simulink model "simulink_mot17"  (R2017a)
settings: Solver=VariableStepAuto  StartTime=0.0  StopTime=1  MaxStep=0.0001  RelTol=1e-5
undefined symbols (not defined in the file or in its folder): j

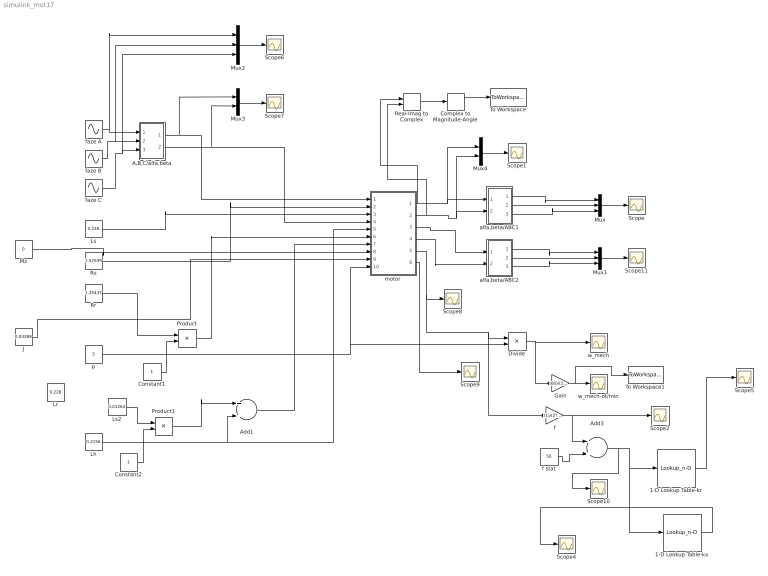
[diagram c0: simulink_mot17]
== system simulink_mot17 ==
  1-D Lookup Table-kr : Lookup_n-D  NumberOfTableDimensions=1  BreakpointsForDimension1="[0\t1.02040816326531\t2.04081632653061\t3.06122448979592\t4.08163265306123\t5.10204081632653\t6.12244897959184\t7.14285714285714\t8.16326530612245\t9.18367346938776\t10.2040816326531\t11.2244897959184\t12.2448979591837\t13.2653061224490\t14.2857142857143\t15.3061224489796\t16.3265306122449\t17.3469387755102\t18.3673469387755\t19.3877551020408\t20.4081632653061\t21.4285714285714\t22.4489795918367\t23.4693877551020\t24.489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"  Table="[1.00000000000000\t1.00003541196316\t1.00014163999465\t1.00031866052521\t1.00056643428835\t1.00088490634371\t1.00127400610982\t1.00173364740605\t1.00226372850387\t1.00286413218725\t1.00353472582216\t1.00427536143518\t1.00508587580093\t1.00596609053850\t1.00691581221651\t1.00793483246685\t1.00902292810692\t1.01017986127023\t1.01140537954524\t1.01269921612228\t1.01406108994838\t1.01549070588984\t1.01698775490243\t1.018551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"  InternalRulePriority=Speed  RndMeth=Simplest
  1-D Lookup Table-kx : Lookup_n-D  NumberOfTableDimensions=1  BreakpointsForDimension1="[0\t1.02040816326531\t2.04081632653061\t3.06122448979592\t4.08163265306123\t5.10204081632653\t6.12244897959184\t7.14285714285714\t8.16326530612245\t9.18367346938776\t10.2040816326531\t11.2244897959184\t12.2448979591837\t13.2653061224490\t14.2857142857143\t15.3061224489796\t16.3265306122449\t17.3469387755102\t18.3673469387755\t19.3877551020408\t20.4081632653061\t21.4285714285714\t22.4489795918367\t23.4693877551020\t24.489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"  Table="[1.00000000000000\t0.999988691005197\t0.999954766683005\t0.999898235018478\t0.999819109314739\t0.999717408185028\t0.999593155541589\t0.999446380581399\t0.999277117768758\t0.999085406814764\t0.998871292653684\t0.998634825416263\t0.998376060399988\t0.998095058036341\t0.997791883855089\t0.997466608445635\t0.997119307415473\t0.996750061345821\t0.996358955744429\t0.995946080995662\t0.995511532307881\t0.995055409658204\t0.99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"  InternalRulePriority=Speed  RndMeth=Simplest
  A,B,C/alfa,beta : Subsystem
  Add1 : Sum
  Add3 : Sum  Inputs=-+
  Complex to Magnitude-Angle : ComplexToMagnitudeAngle
  Constant1 : Constant
  Constant2 : Constant
  Divide : Product  Inputs=*/
  Gain : Gain  Gain=(60)/(2*pi)
  J : Constant  Value=0.03389
  Lh : Constant  Value=0.2156
  Lr : Constant  Value=0.228
  Ls : Constant  Value=0.226
  Ls2 : Constant  Value=0.01264
  Mux : Mux  Inputs=3
  Mux1 : Mux  Inputs=3
  Mux2 : Mux  Inputs=3
  Mux3 : Mux  Inputs=2
  Mux4 : Mux  Inputs=2
  Mz : Constant  Value=0
  Product : Product
  Product1 : Product
  Real-Imag to Complex : RealImagToComplex
  Rr : Constant  Value=1.35437
  Rs : Constant  Value=1.52939
  Scope{,1..2,4..11} (11 alike) : Scope
  To Workspace : ToWorkspace  VariableName=Istat  SampleTime=-1
  To Workspace1 : ToWorkspace  VariableName=ot  SampleTime=-1
  alfa,beta/ABC1 : Subsystem
  alfa,beta/ABC2 : Subsystem
  f : Gain  Gain=(1)/(2*pi)
  f stat : Constant  Value=50
  faze A : Sin  Amplitude=230*1.41421356237309  Frequency=314.159265  SampleTime=0
  faze B : Sin  Amplitude=230*1.41421356237309  Frequency=314.159265  Phase=-(2*pi/3)  SampleTime=0
  faze C : Sin  Amplitude=230*1.41421356237309  Frequency=314.159265  Phase=(2*pi/3)  SampleTime=0
  motor : Subsystem
  p : Constant  Value=3
  w_mech : Scope
  w_mech-ot/min : Scope
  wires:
  faze A/1 -> Mux2/1, A,B,C/alfa,beta/1(In1)
  faze B/1 -> Mux2/2, A,B,C/alfa,beta/2(In2)
  faze C/1 -> Mux2/3, A,B,C/alfa,beta/3(In3)
  A,B,C/alfa,beta/1(Out1) -> Mux3/1, motor/1(Us_alfa)
  Rs/1 -> motor/2(Rs)
  Ls/1 -> motor/3(Ls)
  Lh/1 -> Add1/2, motor/5(Lh)
  motor/3(Ir_alfa1) -> alfa,beta/ABC2/1(Ir_alfa)
  motor/4(Ir_beta) -> alfa,beta/ABC2/2(Ir_beta)
  motor/1(Is_alfa) -> Real-Imag to Complex/1, Mux4/1, alfa,beta/ABC1/1(Is_alfa)
  motor/2(Is_beta) -> Real-Imag to Complex/2, Mux4/2, alfa,beta/ABC1/2(Is_beta)
  A,B,C/alfa,beta/2(Out2) -> Mux3/2, motor/4(Us beta)
  alfa,beta/ABC1/2(Out2) -> Mux/2
  alfa,beta/ABC1/3(Out3) -> Mux/3
  alfa,beta/ABC2/1(Out1) -> Mux1/1
  alfa,beta/ABC2/2(Out2) -> Mux1/2
  alfa,beta/ABC2/3(Out3) -> Mux1/3
  p/1 -> Divide/2, motor/10(p)
  Mz/1 -> motor/8(Mz)
  J/1 -> motor/9(J)
  motor/5(w_el) -> Scope8/1, f/1, Divide/1
  motor/6(M_elmag1) -> Scope9/1
  Divide/1 -> Gain/1, w_mech/1
  alfa,beta/ABC1/1(Out1) -> Mux/1
  Mux/1 -> Scope/1
  Mux1/1 -> Scope11/1
  Mux2/1 -> Scope6/1
  Mux3/1 -> Scope7/1
  Mux4/1 -> Scope1/1
  Gain/1 -> To Workspace1/1, w_mech-ot/min/1
  f stat/1 -> Add3/2
  f/1 -> Scope2/1, Add3/1
  Add3/1 -> Scope10/1, 1-D Lookup Table-kx/1, 1-D Lookup Table-kr/1
  1-D Lookup Table-kr/1 -> Scope5/1
  Rr/1 -> Product/1
  Product/1 -> motor/6(Rr)
  Real-Imag to Complex/1 -> Complex to Magnitude-Angle/1
  Complex to Magnitude-Angle/1 -> To Workspace/1
  Ls2/1 -> Product1/1
  Product1/1 -> Add1/1
  Add1/1 -> motor/7(Lr)
  1-D Lookup Table-kx/1 -> Scope4/1
  Constant2/1 -> Product1/2
  Constant1/1 -> Product/2

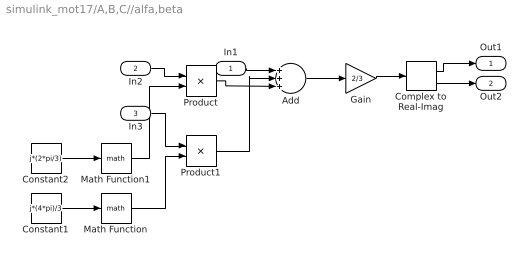
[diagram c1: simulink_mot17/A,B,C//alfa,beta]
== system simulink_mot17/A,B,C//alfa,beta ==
  In1 : Inport
  In2 : Inport  Port=2
  In3 : Inport  Port=3
  Add : Sum  Inputs=+++
  Complex to Real-Imag : ComplexToRealImag
  Constant1 : Constant  Value=j*(4*pi)/3
  Constant2 : Constant  Value=j*(2*pi/3)
  Gain : Gain  Gain=2/3
  Math Function : Math
  Math Function1 : Math
  Product : Product
  Product1 : Product
  Out1 : Outport
  Out2 : Outport  Port=2
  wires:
  Math Function/1 -> Product1/2
  Product1/1 -> Add/2
  Add/1 -> Gain/1
  Constant1/1 -> Math Function/1
  Product/1 -> Add/3
  Complex to Real-Imag/2 -> Out2/1
  Gain/1 -> Complex to Real-Imag/1
  Math Function1/1 -> Product/2
  In3/1 -> Product1/1
  Complex to Real-Imag/1 -> Out1/1
  Constant2/1 -> Math Function1/1
  In1/1 -> Add/1
  In2/1 -> Product/1

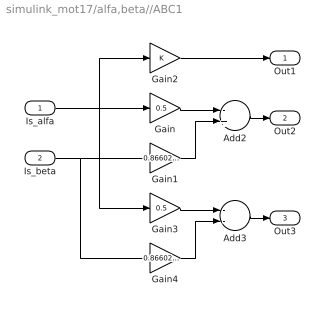
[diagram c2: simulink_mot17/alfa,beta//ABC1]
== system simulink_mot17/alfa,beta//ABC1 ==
  Is_alfa : Inport
  Is_beta : Inport  Port=2
  Add2 : Sum  Inputs=-+
  Add3 : Sum  Inputs=--
  Gain : Gain  Gain=0.5
  Gain1 : Gain  Gain=0.8660254037844
  Gain2 : Gain
  Gain3 : Gain  Gain=0.5
  Gain4 : Gain  Gain=0.8660254037844
  Out1 : Outport
  Out2 : Outport  Port=2
  Out3 : Outport  Port=3
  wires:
  Gain/1 -> Add2/1
  Is_alfa/1 -> Gain3/1, Gain2/1, Gain/1
  Gain4/1 -> Add3/2
  Gain1/1 -> Add2/2
  Is_beta/1 -> Gain4/1, Gain1/1
  Gain3/1 -> Add3/1
  Add2/1 -> Out2/1
  Add3/1 -> Out3/1
  Gain2/1 -> Out1/1

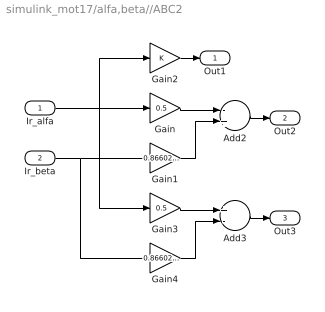
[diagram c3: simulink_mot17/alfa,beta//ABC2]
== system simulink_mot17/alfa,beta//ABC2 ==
  Ir_alfa : Inport
  Ir_beta : Inport  Port=2
  Add2 : Sum  Inputs=-+
  Add3 : Sum  Inputs=+-
  Gain : Gain  Gain=0.5
  Gain1 : Gain  Gain=0.8660254037844
  Gain2 : Gain
  Gain3 : Gain  Gain=0.5
  Gain4 : Gain  Gain=0.8660254037844
  Out1 : Outport
  Out2 : Outport  Port=2
  Out3 : Outport  Port=3
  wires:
  Gain/1 -> Add2/1
  Ir_alfa/1 -> Gain3/1, Gain2/1, Gain/1
  Gain4/1 -> Add3/2
  Gain1/1 -> Add2/2
  Ir_beta/1 -> Gain4/1, Gain1/1
  Gain3/1 -> Add3/1
  Add2/1 -> Out2/1
  Add3/1 -> Out3/1
  Gain2/1 -> Out1/1

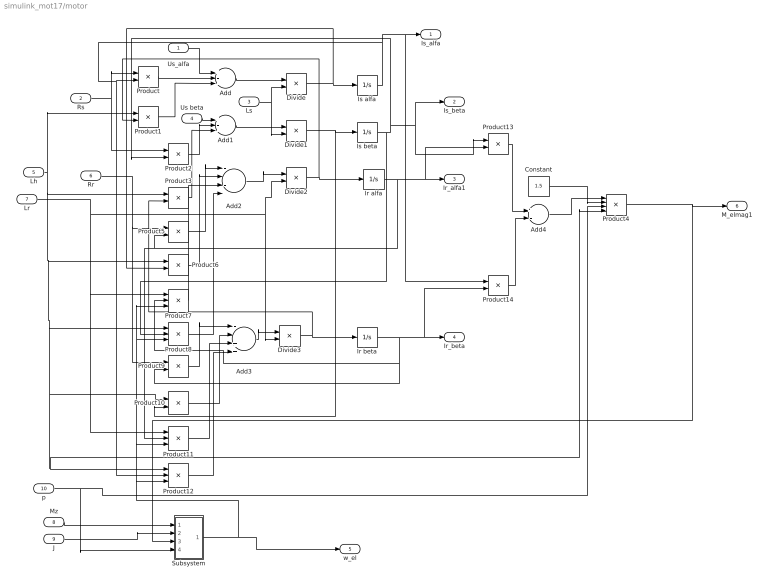
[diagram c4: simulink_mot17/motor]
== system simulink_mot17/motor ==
  Us_alfa : Inport
  Rs : Inport  Port=2
  Ls : Inport  Port=3
  Us beta : Inport  Port=4
  Lh : Inport  Port=5
  Rr : Inport  Port=6
  Lr : Inport  Port=7
  Mz : Inport  Port=8
  J : Inport  Port=9
  p : Inport  Port=10
  Add : Sum  Inputs=+--
  Add1 : Sum  Inputs=+--
  Add2 : Sum  Inputs=----
  Add3 : Sum  Inputs=--++
  Add4 : Sum  Inputs=+-
  Constant : Constant  Value=1.5
  Divide{,1..3} (4 alike) : Product  Inputs=*/
  Ir alfa : Integrator
  Ir beta : Integrator
  Is alfa : Integrator
  Is beta : Integrator
  Product{,1..3,5..6,9..10,13..14} (10 alike) : Product
  Product{7..8,11..12} (4 alike) : Product  Inputs=3
  Product4 : Product  Inputs=4
  Subsystem : Subsystem
  Is_alfa : Outport
  Is_beta : Outport  Port=2
  Ir_alfa1 : Outport  Port=3
  Ir_beta : Outport  Port=4
  w_el : Outport  Port=5
  M_elmag1 : Outport  Port=6
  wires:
  Lh/1 -> Product4/4, Product12/1, Product10/1, Product8/1, Product6/1, Product3/1, Product1/1
  Product6/1 -> Add2/2
  Product8/1 -> Add2/4
  Ir alfa/1 -> Product13/2, Ir_alfa1/1, Product11/2, Product5/2
  Product7/1 -> Add2/3
  Rs/1 -> Product2/1, Product/1
  Product1/1 -> Add/3
  Product/1 -> Add/2
  Is beta/1 -> Is_beta/1, Product13/1, Product2/2, Product8/2
  Ls/1 -> Divide1/2, Divide/2
  Add1/1 -> Divide1/1
  Divide2/1 -> Ir alfa/1, Product1/2
  Add/1 -> Divide/1
  Is alfa/1 -> Product14/1, Is_alfa/1, Product12/2, Product/2
  Product3/1 -> Add1/3
  Add2/1 -> Divide2/1
  Product5/1 -> Add2/1
  Rr/1 -> Product9/1, Product5/1
  Lr/1 -> Product11/1, Product7/1, Divide2/2, Divide3/2
  Product2/1 -> Add1/2
  Us beta/1 -> Add1/1
  Us_alfa/1 -> Add/1
  Product10/1 -> Add3/2
  Product11/1 -> Add3/3
  Divide3/1 -> Ir beta/1, Product3/2
  Product12/1 -> Add3/4
  Divide/1 -> Product6/2, Is alfa/1
  Divide1/1 -> Product10/2, Is beta/1
  Product9/1 -> Add3/1
  Add3/1 -> Divide3/1
  Mz/1 -> Subsystem/1(Mz)
  J/1 -> Subsystem/2(J)
  p/1 -> Subsystem/4(p), Product4/3
  Subsystem/1(Out1) -> Product12/3, Product11/3, Product8/3, Product7/3, w_el/1
  Ir beta/1 -> Product14/2, Ir_beta/1, Product9/2, Product7/2
  Product13/1 -> Add4/1
  Product14/1 -> Add4/2
  Add4/1 -> Product4/1
  Constant/1 -> Product4/2
  Product4/1 -> Subsystem/3(Melmag), M_elmag1/1

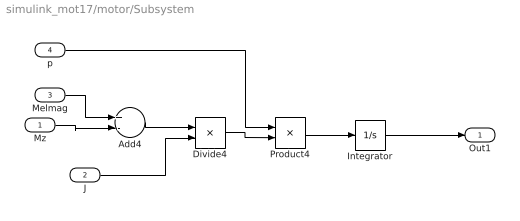
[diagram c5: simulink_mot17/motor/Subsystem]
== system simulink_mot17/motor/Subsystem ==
  Mz : Inport
  J : Inport  Port=2
  Melmag : Inport  Port=3
  p : Inport  Port=4
  Add4 : Sum  Inputs=+-
  Divide4 : Product  Inputs=*/
  Integrator : Integrator
  Product4 : Product
  Out1 : Outport
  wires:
  Melmag/1 -> Add4/1
  Add4/1 -> Divide4/1
  Integrator/1 -> Out1/1
  p/1 -> Product4/1
  Product4/1 -> Integrator/1
  J/1 -> Divide4/2
  Mz/1 -> Add4/2
  Divide4/1 -> Product4/2
